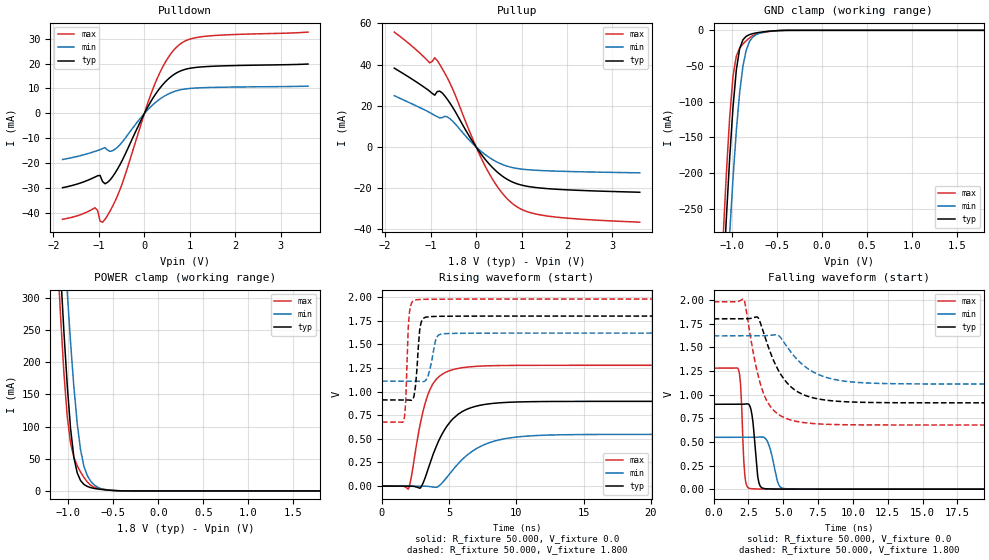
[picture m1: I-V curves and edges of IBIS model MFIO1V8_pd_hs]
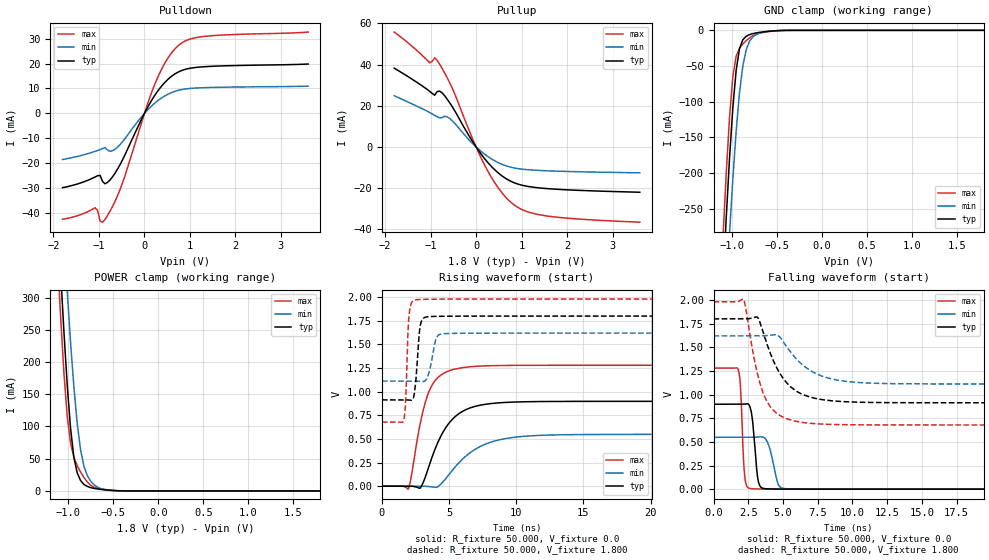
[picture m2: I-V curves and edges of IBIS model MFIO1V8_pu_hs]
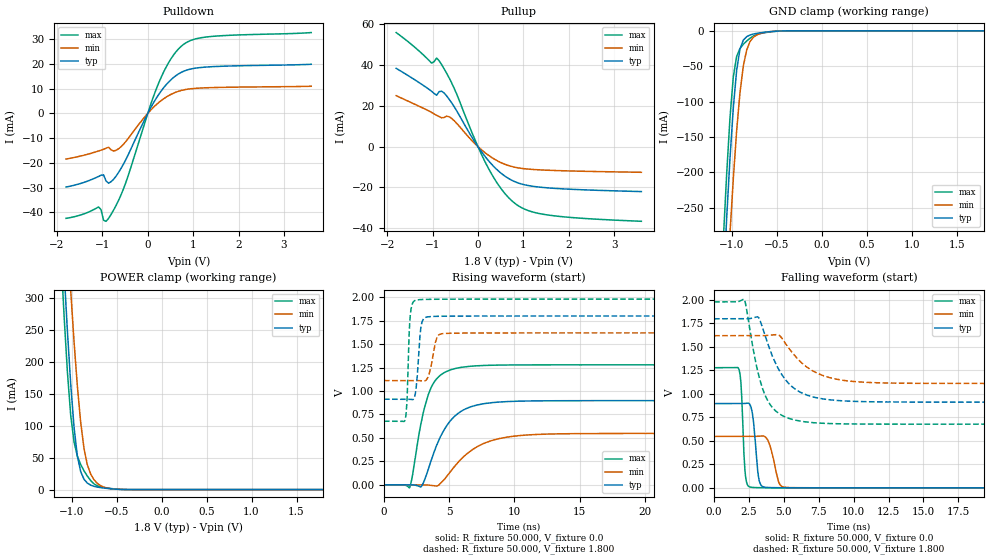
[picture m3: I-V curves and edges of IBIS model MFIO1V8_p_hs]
| IBIS file lpc55s6x_htqfp64.ibs
[IBIS Ver]   5.0
[File name]   lpc55s6x_htqfp64.ibs
[File Rev]   1.0
[Date]   June 05,2020
[Notes]   Rev History
|   1.0  initial release
[Disclaimer]   The model given below represents a 64-pin package.
[Copyright]   Copyright NXP 2020
[Component] lpc55s6x
[Manufacturer] NXP
[Package]
|   typ   min   max
R_pkg   0.17989   0.11672   0.21665
L_pkg   3.582e-9   2.713e-9   4.471e-9
C_pkg   5.658e-13   4.885e-13   6.682e-13
[Pin]   Signal_name   model_name   R_pin   L_pin   C_pin
32   VBAT_DCDC   POWER   NA   NA   NA
33   VBAT_PMU   POWER   NA   NA   NA
25   VBUS   POWER   NA   NA   NA
9   VDDA   POWER   NA   NA   NA
27   USB1_3V3   POWER   NA   NA   NA
61   USB0_3V3   POWER   NA   NA   NA
8   VDD   POWER   NA   NA   NA
16   VDD   POWER   NA   NA   NA
43   VDD   POWER   NA   NA   NA
54   VDD   POWER   NA   NA   NA
28   VDD_PMU   POWER   NA   NA   NA
11   VSSA   POWER   NA   NA   NA
10   VREFP   POWER   NA   NA   NA
24   USB1_DM   NC   0.17504   3.032e-9   5.223e-13
23   USB1_DP   NC   0.17514   3.092e-9   5.851e-13
29   FB   NC   0.17997   3.2e-9   5.501e-13
31   LX   NC   0.11672   2.713e-9   6.682e-13
36   P0_0   gpio1v8   0.16617   3.518e-9   5.45e-13
2   P0_1   gpio1v8   0.21061   4.26e-9   6.597e-13
52   P0_2   gpio1v8   0.17565   3.663e-9   5.472e-13
53   P0_3   gpio1v8   0.18057   3.358e-9   5.428e-13
55   P0_4   gpio1v8   0.17327   3.383e-9   5.051e-13
56   P0_5   gpio1v8   0.16709   3.405e-9   5.309e-13
57   P0_6   gpio1v8   0.16522   3.425e-9   5.279e-13
1   P0_7   gpio1v8   0.21665   4.471e-9   5.383e-13
17   P0_8   gpio1v8   0.18848   4.018e-9   5.105e-13
37   P0_9   gpio1v8   0.16187   3.431e-9   5.312e-13
13   P0_10   gpio1v8   0.17253   3.573e-9   5.676e-13
6   P0_11   gpio1v8   0.18173   3.605e-9   5.495e-13
5   P0_12   gpio1v8   0.19018   3.808e-9   5.757e-13
46   P0_13   iicgpio1v8   0.1835   3.808e-9   6.094e-13
47   P0_14   iicgpio1v8   0.19388   3.993e-9   6.262e-13
14   P0_15   gpio1v8   0.18145   3.701e-9   6.007e-13
7   P0_16   gpio1v8   0.17986   3.266e-9   6.176e-13
3   P0_17   gpio1v8   0.19764   4.058e-9   6.393e-13
38   P0_18   gpio1v8   0.16061   3.395e-9   5.068e-13
58   P0_19   gpio1v8   0.16651   3.498e-9   6.032e-13
48   P0_20   gpio1v8   0.1987   4.192e-9   5.125e-13
49   P0_21   gpio1v8   0.18929   4.138e-9   5.17e-13
50   P0_22   gpio1v8   0.18233   3.903e-9   5.815e-13
12   P0_23   gpio1v8   0.1715   3.281e-9   5.416e-13
45   P0_24   gpio1v8   0.17483   3.63e-9   5.425e-13
51   P0_25   gpio1v8   0.17633   3.765e-9   5.604e-13
40   P0_26   gpio1v8   0.16354   3.315e-9   5.176e-13
18   P0_27   gpio1v8   0.17719   3.735e-9   6.145e-13
44   P0_28   gpio1v8   0.193   3.536e-9   5.322e-13
59   P0_29   gpio1v8   0.16968   3.503e-9   5.331e-13
60   P0_30   gpio1v8   0.1805   3.361e-9   5.439e-13
15   P0_31   gpio1v8   0.19849   3.721e-9   6.033e-13
4   P1_0   gpio1v8   0.20125   4.033e-9   5.79e-13
39   P1_1   gpio1v8   0.16081   3.349e-9   4.885e-13
41   P1_2   gpio1v8   0.17007   3.348e-9   5.264e-13
42   P1_3   gpio1v8   0.18622   3.305e-9   5.922e-13
21   RESETN   gpio1v8   0.18027   3.291e-9   5.21e-13
63   USB0_DM   NC   0.2064   3.561e-9   6.583e-13
62   USB0_DP   NC   0.19683   3.467e-9   6.489e-13
35   XTAL32K_N   NC   0.1734   3.529e-9   5.779e-13
34   XTAL32K_P   NC   0.19207   3.472e-9   5.963e-13
19   XTAL32M_N   NC   0.1793   3.701e-9   6.074e-13
20   XTAL32M_P   NC   0.17246   3.538e-9   5.342e-13
65   VSS   GND   NA   NA   NA
22   USB1_VSS   GND   NA   NA   NA
26   USB1_VSS   GND   NA   NA   NA
30   VSS_DCDC   GND   NA   NA   NA
64   USB0_VSS   GND   NA   NA   NA
|   Model Selector
[Model Selector] gpio1v8
MFIO1V8_pd_hs  EPUN=1 EPD=1 EHS=1
MFIO1V8_pd_ls  EPUN=1 EPD=1 EHS=0
MFIO1V8_pu_hs  EPUN=0 EPD=0 EHS=1
MFIO1V8_pu_ls  EPUN=0 EPD=0 EHS=0
MFIO1V8_p_hs  EPUN=1 EPD=0 EHS=1
MFIO1V8_p_ls  EPUN=1 EPD=0 EHS=0
MFIO1V8_r_hs  EPUN=0 EPD=1 EHS=1
MFIO1V8_r_ls  EPUN=0 EPD=1 EHS=0
[Model Selector] iicgpio1v8
IIC1V8_pd_hs  EGP=1 EPUN=1 EPD=1 EHS=1
IIC1V8_pd_ls  EGP=1 EPUN=1 EPD=1 EHS=0
IIC1V8_p_hs  EGP=1 EPUN=1 EPD=0 EHS=1
IIC1V8_p_ls  EGP=1 EPUN=1 EPD=0 EHS=0
IIC1V8_pu_hs  EGP=1 EPUN=0 EPD=0 EHS=1
IIC1V8_pu_ls  EGP=1 EPUN=0 EPD=0 EHS=0
IIC1V8_r_hs  EGP=1 EPUN=0 EPD=1 EHS=1
IIC1V8_r_ls  EGP=1 EPUN=0 EPD=1 EHS=0
IIC1V8_pd_iic_hs  EGP=0 ECS=0 EPUN=1 EPD=1
IIC1V8_p_iic_hs  EGP=0 ECS=0 EPUN=1 EPD=0
IIC1V8_pu_iic_hs  EGP=0 ECS=0 EPUN=0 EPD=0
IIC1V8_r_iic_hs  EGP=0 ECS=0 EPUN=0 EPD=1
IIC1V8_pd_iic_pu_hs  EGP=0 ECS=1 EPUN=1 EPD=1  SSEL=1
IIC1V8_p_iic_pu_hs  EGP=0 ECS=1 EPUN=1 EPD=0  SSEL=1
IIC1V8_pu_iic_pu_hs  EGP=0 ECS=1 EPUN=0 EPD=0  SSEL=1
IIC1V8_r_iic_pu_hs  EGP=0 ECS=1 EPUN=0 EPD=1  SSEL=1
| Models and submodels in the file (24): MFIO1V8_pd_hs (I/O), MFIO1V8_pd_ls (I/O), MFIO1V8_pu_hs (I/O), MFIO1V8_pu_ls (I/O), MFIO1V8_p_hs (I/O), MFIO1V8_p_ls (I/O), MFIO1V8_r_hs (I/O), MFIO1V8_r_ls (I/O), IIC1V8_pd_hs (I/O), IIC1V8_pd_ls (I/O), IIC1V8_p_hs (I/O), IIC1V8_p_ls (I/O), IIC1V8_pu_hs (I/O), IIC1V8_pu_ls (I/O), IIC1V8_r_hs (I/O), IIC1V8_r_ls (I/O), IIC1V8_pd_iic_hs (I/O_open_drain), IIC1V8_p_iic_hs (I/O_open_drain), IIC1V8_pu_iic_hs (I/O_open_drain), IIC1V8_r_iic_hs (I/O_open_drain), IIC1V8_pd_iic_pu_hs (I/O_open_drain), IIC1V8_p_iic_pu_hs (I/O_open_drain), IIC1V8_pu_iic_pu_hs (I/O_open_drain), IIC1V8_r_iic_pu_hs (I/O_open_drain)
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|   Model MFIO1V8_pd_hs
[Model] MFIO1V8_pd_hs
Model_type I/O
Polarity   Non-Inverting
Enable   Active-Low
Vinl =  0.540V
Vinh =  1.260V
Vmeas =  0.900V
Cref =  0.0F
Rref =  100.000
Vref =  0.0V
C_comp   2.019pF   1.989pF   2.068pF
C_comp_pullup   1.198pF   1.161pF   1.251pF
C_comp_pulldown   0.670pF   0.661pF   0.684pF
[Model Spec]
Vinh   1.260V   1.134V   1.386V
Vinl   0.540V   0.486V   0.594V
Vmeas   0.900V   0.810V   0.990V
Vref   0.0V   0.0V   0.0V
Cref   0.0F   0.0F   0.0F
Rref   100.000   100.000   100.000
[Temperature Range]   25.000   0.125k   -40.000
[Voltage Range]   1.800V   1.620V   1.980V
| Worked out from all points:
|   slope of the pulldown table from 0 to 0.27 V, typ, clamps not added: 32.2 ohm
|   slope of the pullup table from 0 to 0.27 V, typ, clamps not added: 34.3 ohm
|   GND clamp passes 1 mA (typ) near -0.56 V on its own axis
|   POWER clamp passes 1 mA (typ) near -0.54 V on its own axis
|   rising waveform, R_fixture 50.000, V_fixture 0.0: 20-80 % time 1.89ns typ, 2.69ns min, 1.21ns max; typ from 0 V to 0.897 V
|   rising waveform, R_fixture 50.000, V_fixture 1.800: 20-80 % time 276ps typ, 422ps min, 194ps max; typ from 0.912 V to 1.8 V
|   falling waveform, R_fixture 50.000, V_fixture 0.0: 20-80 % time 315ps typ, 502ps min, 217ps max; typ from 0.897 V to 0 V
|   falling waveform, R_fixture 50.000, V_fixture 1.800: 20-80 % time 1.84ns typ, 2.3ns min, 1.28ns max; typ from 1.8 V to 0.912 V
[Pulldown]
|Voltage   I(typ)   I(min)   I(max)
-1.8V     -29.75mA   -18.45mA   -42.39mA
-1.085V   -25.48mA   -15.2mA    -37.79mA
-1.03V    -24.99mA   -14.87mA   -38.88mA
-975mV    -24.83mA   -14.51mA   -43.15mA
-865mV    -28.18mA   -13.68mA   -42.43mA
-700mV    -25.38mA   -14.92mA   -37.23mA
-480mV    -18.54mA   -11.29mA   -27.73mA
235mV     7.474mA    4.265mA    12.03mA
510mV     13.55mA    7.648mA    22.01mA
785mV     16.96mA    9.446mA    27.8mA
1.39V     18.81mA    10.38mA    31.01mA
3.6V      19.8mA     10.93mA    32.61mA
[Pullup]
|Voltage   I(typ)   I(min)   I(max)
-1.8V     38.29mA    24.9mA     55.82mA
-1.02V    27.05mA    16.71mA    40.87mA
-910mV    25.14mA    15.31mA    43.32mA
-855mV    26.89mA    14.69mA    42.04mA
-745mV    26.24mA    14.22mA    38.06mA
-580mV    21.45mA    13.82mA    31.22mA
190mV     -5.761mA   -3.564mA   -8.914mA
520mV     -13.24mA   -7.997mA   -20.92mA
795mV     -17.02mA   -10.03mA   -27.47mA
1.07V     -18.92mA   -10.95mA   -31.04mA
1.51V     -20.18mA   -11.56mA   -33.41mA
3.6V      -22.04mA   -12.6mA    -36.6mA
[GND_clamp]
|Voltage   I(typ)   I(min)   I(max)
-1.8V     -2.463A    -2.494A    -2.446A
-1.097V   -357.7mA   -460.7mA   -294.8mA
-1.06V    -264.9mA   -370.9mA   -202.5mA
-1.023V   -180.4mA   -286.3mA   -122.9mA
-986mV    -108.7mA   -208.9mA   -65.05mA
-949mV    -56.06mA   -141.4mA   -36.24mA
-912mV    -25.87mA   -87.65mA   -25.01mA
-875mV    -13.21mA   -49.99mA   -19.06mA
-838mV    -8.315mA   -27.44mA   -14.52mA
-764mV    -4.558mA   -9.219mA   -7.395mA
-542mV    -813.9uA   -810.7uA   -1.086mA
1.8V      0A         0A         0A
[POWER_clamp]
|Voltage   I(typ)   I(min)   I(max)
-1.8V     2.577A     2.626A     2.553A
-1.123V   442.8mA    582.7mA    371.8mA
-1.086V   342mA      487.8mA    272.2mA
-1.049V   248.2mA    396.7mA    184.1mA
-1.012V   164.7mA    310.5mA    115.9mA
-975mV    97.4mA     231.2mA    74.47mA
-938mV    52.21mA    161.5mA    52.2mA
-864mV    16.15mA    64.06mA    29.43mA
-790mV    7.073mA    24.26mA    14.23mA
-679mV    3.152mA    6.087mA    4.407mA
-494mV    590.1uA    655.5uA    758.5uA
1.8V      0A         0A         0A
[Ramp]
| variable   typ   min   max
dV/dt_r   0.538/1.890n   0.328/2.680n   0.767/1.209n
dV/dt_f   0.532/1.835n   0.305/2.291n   0.781/1.275n
R_load = 50.000
[Rising Waveform]
R_fixture= 50.000
V_fixture= 0.0
V_fixture_min= 0.0
V_fixture_max= 0.0
|time   V(typ)   V(min)   V(max)
0s        6.721nV    117.6nV    4.416nV
1.96ns    159.2uV    -62.09nV   -31.69mV
2.85ns    -21.07mV   134.7uV    661mV
3.65ns    271.3mV    -6.708mV   1.047V
4.15ns    457.1mV    -8.65mV    1.146V
4.97ns    661.3mV    117.8mV    1.218V
6.65ns    830.9mV    361.7mV    1.264V
9.15ns    884.8mV    501.2mV    1.276V
13.74ns   896.1mV    543.8mV    1.278V
100ns     896.7mV    547.4mV    1.278V
[Rising Waveform]
R_fixture= 50.000
V_fixture= 1.800
V_fixture_min= 1.620
V_fixture_max= 1.980
|time   V(typ)   V(min)   V(max)
0s        911.9mV    1.111V     677.7mV
1.63ns    911.9mV    1.111V     697.7mV
1.77ns    912.1mV    1.111V     900.3mV
2.05ns    909.6mV    1.111V     1.849V
2.42ns    983.6mV    1.111V     1.967V
2.68ns    1.419V     1.11V      1.973V
3.06ns    1.772V     1.105V     1.976V
4.08ns    1.796V     1.575V     1.978V
4.84ns    1.798V     1.614V     1.979V
100ns     1.799V     1.619V     1.979V
[Falling Waveform]
R_fixture= 50.000
V_fixture= 0.0
V_fixture_min= 0.0
V_fixture_max= 0.0
|time   V(typ)   V(min)   V(max)
0s        896.7mV    547.4mV    1.278V
1.79ns    896.7mV    547.4mV    1.258V
1.93ns    896.6mV    547.4mV    1.106V
2.24ns    898.4mV    547.4mV    142.2mV
2.74ns    796.7mV    547.3mV    4.509mV
3.2ns     100.7mV    550.1mV    1.658mV
3.81ns    3.552mV    517mV      778.9uV
4.65ns    1.171mV    54.78mV    345.8uV
5.34ns    645.9uV    3.088mV    186.5uV
100ns     14.3nV     131.2nV    8.877nV
[Falling Waveform]
R_fixture= 50.000
V_fixture= 1.800
V_fixture_min= 1.620
V_fixture_max= 1.980
|time   V(typ)   V(min)   V(max)
0s        1.799V     1.619V     1.979V
2.17ns    1.799V     1.619V     2.003V
3.18ns    1.813V     1.619V     1.21V
3.88ns    1.522V     1.623V     915.7mV
4.62ns    1.262V     1.626V     793.3mV
5.16ns    1.14V      1.527V     750mV
6.98ns    971mV      1.252V     694.9mV
9.25ns    925.2mV    1.144V     680.9mV
13.25ns   913mV      1.113V     677.9mV
100ns     911.9mV    1.111V     677.7mV
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|   Model MFIO1V8_pu_hs
[Model] MFIO1V8_pu_hs
Model_type I/O
Polarity   Non-Inverting
Enable   Active-Low
Vinl =  0.540V
Vinh =  1.260V
Vmeas =  0.900V
Cref =  0.0F
Rref =  100.000
Vref =  0.0V
C_comp   2.019pF   1.989pF   2.068pF
C_comp_pullup   1.197pF   1.159pF   1.249pF
C_comp_pulldown   0.671pF   0.662pF   0.686pF
[Model Spec]
Vinh   1.260V   1.134V   1.386V
Vinl   0.540V   0.486V   0.594V
Vmeas   0.900V   0.810V   0.990V
Vref   0.0V   0.0V   0.0V
Cref   0.0F   0.0F   0.0F
Rref   100.000   100.000   100.000
[Temperature Range]   25.000   0.125k   -40.000
[Voltage Range]   1.800V   1.620V   1.980V
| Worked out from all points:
|   slope of the pulldown table from 0 to 0.27 V, typ, clamps not added: 32.2 ohm
|   slope of the pullup table from 0 to 0.27 V, typ, clamps not added: 34.3 ohm
|   GND clamp passes 1 mA (typ) near -0.56 V on its own axis
|   POWER clamp passes 1 mA (typ) near -0.54 V on its own axis
|   rising waveform, R_fixture 50.000, V_fixture 0.0: 20-80 % time 1.89ns typ, 2.68ns min, 1.21ns max; typ from 0.001 V to 0.898 V
|   rising waveform, R_fixture 50.000, V_fixture 1.800: 20-80 % time 275ps typ, 425ps min, 197ps max; typ from 0.913 V to 1.8 V
|   falling waveform, R_fixture 50.000, V_fixture 0.0: 20-80 % time 314ps typ, 505ps min, 216ps max; typ from 0.898 V to 0.001 V
|   falling waveform, R_fixture 50.000, V_fixture 1.800: 20-80 % time 1.84ns typ, 2.3ns min, 1.27ns max; typ from 1.8 V to 0.913 V
[Pulldown]
|Voltage   I(typ)   I(min)   I(max)
-1.8V     -29.75mA   -18.45mA   -42.39mA
-1.085V   -25.48mA   -15.2mA    -37.79mA
-1.03V    -24.99mA   -14.87mA   -38.88mA
-975mV    -24.83mA   -14.51mA   -43.15mA
-865mV    -28.18mA   -13.68mA   -42.43mA
-700mV    -25.38mA   -14.92mA   -37.23mA
-480mV    -18.54mA   -11.29mA   -27.73mA
235mV     7.474mA    4.265mA    12.03mA
510mV     13.55mA    7.648mA    22.01mA
785mV     16.96mA    9.446mA    27.8mA
1.39V     18.81mA    10.38mA    31.01mA
3.6V      19.8mA     10.93mA    32.61mA
[Pullup]
|Voltage   I(typ)   I(min)   I(max)
-1.8V     38.29mA    24.9mA     55.82mA
-1.02V    27.05mA    16.71mA    40.87mA
-910mV    25.14mA    15.31mA    43.32mA
-855mV    26.89mA    14.69mA    42.04mA
-745mV    26.24mA    14.22mA    38.06mA
-580mV    21.45mA    13.82mA    31.22mA
190mV     -5.761mA   -3.564mA   -8.914mA
520mV     -13.24mA   -7.997mA   -20.92mA
795mV     -17.02mA   -10.03mA   -27.47mA
1.07V     -18.92mA   -10.95mA   -31.04mA
1.51V     -20.18mA   -11.56mA   -33.41mA
3.6V      -22.04mA   -12.6mA    -36.6mA
[GND_clamp]
|Voltage   I(typ)   I(min)   I(max)
-1.8V     -2.463A    -2.494A    -2.446A
-1.097V   -357.7mA   -460.7mA   -294.9mA
-1.06V    -264.9mA   -371mA     -202.6mA
-1.023V   -180.4mA   -286.4mA   -122.9mA
-986mV    -108.7mA   -208.9mA   -65.09mA
-949mV    -56.09mA   -141.5mA   -36.28mA
-912mV    -25.91mA   -87.68mA   -25.06mA
-875mV    -13.24mA   -50.02mA   -19.11mA
-838mV    -8.35mA    -27.47mA   -14.57mA
-764mV    -4.593mA   -9.247mA   -7.441mA
-542mV    -849.5uA   -838.5uA   -1.132mA
1.8V      0A         0A         0A
[POWER_clamp]
|Voltage   I(typ)   I(min)   I(max)
-1.8V     2.577A     2.626A     2.553A
-1.123V   442.8mA    582.7mA    371.7mA
-1.086V   342mA      487.8mA    272.2mA
-1.049V   248.2mA    396.7mA    184.1mA
-1.012V   164.7mA    310.5mA    115.9mA
-975mV    97.36mA    231.1mA    74.42mA
-938mV    52.18mA    161.5mA    52.15mA
-864mV    16.11mA    64.03mA    29.39mA
-790mV    7.037mA    24.23mA    14.18mA
-679mV    3.116mA    6.059mA    4.361mA
-494mV    554.4uA    627.7uA    712.3uA
1.8V      0A         0A         0A
[Ramp]
| variable   typ   min   max
dV/dt_r   0.538/1.890n   0.329/2.680n   0.767/1.209n
dV/dt_f   0.532/1.835n   0.305/2.290n   0.781/1.276n
R_load = 50.000
[Rising Waveform]
R_fixture= 50.000
V_fixture= 0.0
V_fixture_min= 0.0
V_fixture_max= 0.0
|time   V(typ)   V(min)   V(max)
0s        630.6uV    679.1uV    587.5uV
1.96ns    789.2uV    678.8uV    -30.05mV
2.85ns    -19.7mV    812.3uV    661.1mV
3.62ns    261mV      -5.421mV   1.04V
4.13ns    453.5mV    -9.012mV   1.145V
4.91ns    652mV      107.5mV    1.216V
6.6ns     829.9mV    358mV      1.264V
9.06ns    885.4mV    500.2mV    1.277V
13.76ns   897.4mV    545.1mV    1.28V
100ns     898mV      548.7mV    1.28V
[Rising Waveform]
R_fixture= 50.000
V_fixture= 1.800
V_fixture_min= 1.620
V_fixture_max= 1.980
|time   V(typ)   V(min)   V(max)
0s        913.3mV    1.112V     678.9mV
1.63ns    913.3mV    1.112V     698.4mV
1.75ns    913.5mV    1.112V     853.9mV
2.02ns    911.7mV    1.112V     1.814V
2.4ns     967.4mV    1.112V     1.968V
2.67ns    1.397V     1.111V     1.974V
3.06ns    1.773V     1.107V     1.977V
4.07ns    1.797V     1.574V     1.979V
4.83ns    1.798V     1.615V     1.98V
100ns     1.8V       1.62V      1.98V
[Falling Waveform]
R_fixture= 50.000
V_fixture= 0.0
V_fixture_min= 0.0
V_fixture_max= 0.0
|time   V(typ)   V(min)   V(max)
0s        898mV      548.7mV    1.28V
1.79ns    898mV      548.7mV    1.259V
1.93ns    897.9mV    548.6mV    1.108V
2.24ns    899.8mV    548.7mV    143.9mV
2.76ns    775.9mV    548.5mV    5.275mV
3.23ns    78.56mV    551.7mV    2.369mV
3.84ns    4.35mV     511.3mV    1.439mV
4.67ns    1.941mV    48.66mV    967uV
5.32ns    1.374mV    4.206mV    798.7uV
100ns     630.7uV    679.1uV    587.5uV
[Falling Waveform]
R_fixture= 50.000
V_fixture= 1.800
V_fixture_min= 1.620
V_fixture_max= 1.980
|time   V(typ)   V(min)   V(max)
0s        1.8V       1.62V      1.98V
2.16ns    1.8V       1.62V      2.006V
3.18ns    1.814V     1.62V      1.212V
3.84ns    1.538V     1.623V     928.3mV
4.62ns    1.264V     1.627V     794.8mV
5.16ns    1.142V     1.528V     751.1mV
7.03ns    970.5mV    1.249V     695.5mV
9.17ns    927.3mV    1.147V     682.3mV
13.26ns   914.4mV    1.115V     679mV
100ns     913.3mV    1.112V     678.9mV
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|   Model MFIO1V8_p_hs
[Model] MFIO1V8_p_hs
Model_type I/O
Polarity   Non-Inverting
Enable   Active-Low
Vinl =  0.540V
Vinh =  1.260V
Vmeas =  0.900V
Cref =  0.0F
Rref =  100.000
Vref =  0.0V
C_comp   2.019pF   1.989pF   2.068pF
C_comp_pullup   1.197pF   1.160pF   1.250pF
C_comp_pulldown   0.671pF   0.662pF   0.686pF
[Model Spec]
Vinh   1.260V   1.134V   1.386V
Vinl   0.540V   0.486V   0.594V
Vmeas   0.900V   0.810V   0.990V
Vref   0.0V   0.0V   0.0V
Cref   0.0F   0.0F   0.0F
Rref   100.000   100.000   100.000
[Temperature Range]   25.000   0.125k   -40.000
[Voltage Range]   1.800V   1.620V   1.980V
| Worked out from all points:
|   slope of the pulldown table from 0 to 0.27 V, typ, clamps not added: 32.2 ohm
|   slope of the pullup table from 0 to 0.27 V, typ, clamps not added: 34.3 ohm
|   GND clamp passes 1 mA (typ) near -0.56 V on its own axis
|   POWER clamp passes 1 mA (typ) near -0.54 V on its own axis
|   rising waveform, R_fixture 50.000, V_fixture 0.0: 20-80 % time 1.89ns typ, 2.68ns min, 1.21ns max; typ from 0 V to 0.897 V
|   rising waveform, R_fixture 50.000, V_fixture 1.800: 20-80 % time 278ps typ, 422ps min, 192ps max; typ from 0.913 V to 1.8 V
|   falling waveform, R_fixture 50.000, V_fixture 0.0: 20-80 % time 314ps typ, 511ps min, 215ps max; typ from 0.897 V to 0 V
|   falling waveform, R_fixture 50.000, V_fixture 1.800: 20-80 % time 1.84ns typ, 2.3ns min, 1.28ns max; typ from 1.8 V to 0.913 V
[Pulldown]
|Voltage   I(typ)   I(min)   I(max)
-1.8V     -29.75mA   -18.45mA   -42.39mA
-1.085V   -25.48mA   -15.2mA    -37.79mA
-1.03V    -24.99mA   -14.87mA   -38.88mA
-975mV    -24.83mA   -14.51mA   -43.15mA
-865mV    -28.18mA   -13.68mA   -42.43mA
-700mV    -25.38mA   -14.92mA   -37.23mA
-480mV    -18.54mA   -11.29mA   -27.73mA
235mV     7.474mA    4.265mA    12.03mA
510mV     13.55mA    7.648mA    22.01mA
785mV     16.96mA    9.446mA    27.8mA
1.39V     18.81mA    10.38mA    31.01mA
3.6V      19.8mA     10.93mA    32.61mA
[Pullup]
|Voltage   I(typ)   I(min)   I(max)
-1.8V     38.29mA    24.9mA     55.82mA
-1.02V    27.05mA    16.71mA    40.87mA
-910mV    25.14mA    15.31mA    43.32mA
-855mV    26.89mA    14.69mA    42.04mA
-745mV    26.24mA    14.22mA    38.06mA
-580mV    21.45mA    13.82mA    31.22mA
190mV     -5.761mA   -3.564mA   -8.914mA
520mV     -13.24mA   -7.997mA   -20.92mA
795mV     -17.02mA   -10.03mA   -27.47mA
1.07V     -18.92mA   -10.95mA   -31.04mA
1.51V     -20.18mA   -11.56mA   -33.41mA
3.6V      -22.04mA   -12.6mA    -36.6mA
[GND_clamp]
|Voltage   I(typ)   I(min)   I(max)
-1.8V     -2.463A    -2.494A    -2.446A
-1.097V   -357.7mA   -460.7mA   -294.8mA
-1.06V    -264.9mA   -370.9mA   -202.5mA
-1.023V   -180.4mA   -286.3mA   -122.9mA
-986mV    -108.6mA   -208.9mA   -65.04mA
-949mV    -56.05mA   -141.4mA   -36.22mA
-912mV    -25.86mA   -87.64mA   -25mA
-875mV    -13.2mA    -49.98mA   -19.05mA
-838mV    -8.305mA   -27.43mA   -14.51mA
-764mV    -4.549mA   -9.211mA   -7.385mA
-542mV    -805.6uA   -803.8uA   -1.077mA
1.8V      0A         0A         0A
[POWER_clamp]
|Voltage   I(typ)   I(min)   I(max)
-1.8V     2.577A     2.626A     2.553A
-1.123V   442.8mA    582.7mA    371.7mA
-1.086V   342mA      487.8mA    272.1mA
-1.049V   248.2mA    396.6mA    184.1mA
-1.012V   164.7mA    310.5mA    115.9mA
-975mV    97.36mA    231.1mA    74.41mA
-938mV    52.17mA    161.5mA    52.14mA
-864mV    16.1mA     64.02mA    29.38mA
-790mV    7.028mA    24.22mA    14.17mA
-679mV    3.108mA    6.053mA    4.351mA
-494mV    546.6uA    621.4uA    702.9uA
1.8V      0A         0A         0A
[Ramp]
| variable   typ   min   max
dV/dt_r   0.538/1.892n   0.329/2.683n   0.768/1.210n
dV/dt_f   0.532/1.838n   0.305/2.294n   0.781/1.277n
R_load = 50.000
[Rising Waveform]
R_fixture= 50.000
V_fixture= 0.0
V_fixture_min= 0.0
V_fixture_max= 0.0
|time   V(typ)   V(min)   V(max)
0s        7.051nV    120nV      4.667nV
1.96ns    159.3uV    -60nV      -31.77mV
2.85ns    -21.07mV   134.7uV    659.8mV
3.66ns    277.4mV    -6.745mV   1.05V
4.15ns    457.5mV    -8.707mV   1.146V
5.02ns    670.7mV    126mV      1.221V
6.67ns    832.3mV    364.4mV    1.265V
9.24ns    886mV      503.8mV    1.277V
13.74ns   896.7mV    544.2mV    1.279V
100ns     897.3mV    547.8mV    1.279V
[Rising Waveform]
R_fixture= 50.000
V_fixture= 1.800
V_fixture_min= 1.620
V_fixture_max= 1.980
|time   V(typ)   V(min)   V(max)
0s        912.6mV    1.112V     678.1mV
1.63ns    912.6mV    1.112V     697.9mV
1.77ns    912.8mV    1.112V     903.5mV
2.03ns    910.9mV    1.112V     1.828V
2.4ns     967.2mV    1.112V     1.967V
2.66ns    1.375V     1.111V     1.974V
3ns       1.761V     1.107V     1.977V
4.06ns    1.797V     1.57V      1.979V
4.83ns    1.798V     1.615V     1.979V
100ns     1.8V       1.62V      1.98V
[Falling Waveform]
R_fixture= 50.000
V_fixture= 0.0
V_fixture_min= 0.0
V_fixture_max= 0.0
|time   V(typ)   V(min)   V(max)
0s        897.3mV    547.8mV    1.279V
1.79ns    897.3mV    547.8mV    1.258V
1.96ns    897.2mV    547.8mV    1.035V
2.25ns    899.3mV    547.8mV    128.7mV
2.75ns    785.4mV    547.7mV    4.896mV
3.23ns    77.6mV     550.8mV    1.878mV
3.83ns    3.769mV    511.9mV    959.3uV
4.67ns    1.371mV    47.13mV    456uV
5.37ns    779.8uV    3.194mV    261.7uV
100ns     14.63nV    133.6nV    9.13nV
[Falling Waveform]
R_fixture= 50.000
V_fixture= 1.800
V_fixture_min= 1.620
V_fixture_max= 1.980
|time   V(typ)   V(min)   V(max)
0s        1.8V       1.62V      1.98V
2.16ns    1.8V       1.62V      2.006V
3.19ns    1.813V     1.62V      1.204V
3.83ns    1.543V     1.623V     931.6mV
4.63ns    1.261V     1.626V     793.3mV
5.2ns     1.135V     1.52V      748.4mV
7.09ns    968mV      1.244V     694.1mV
9.25ns    926.1mV    1.145V     681.3mV
13.38ns   913.7mV    1.114V     678.3mV
100ns     912.6mV    1.112V     678.1mV
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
